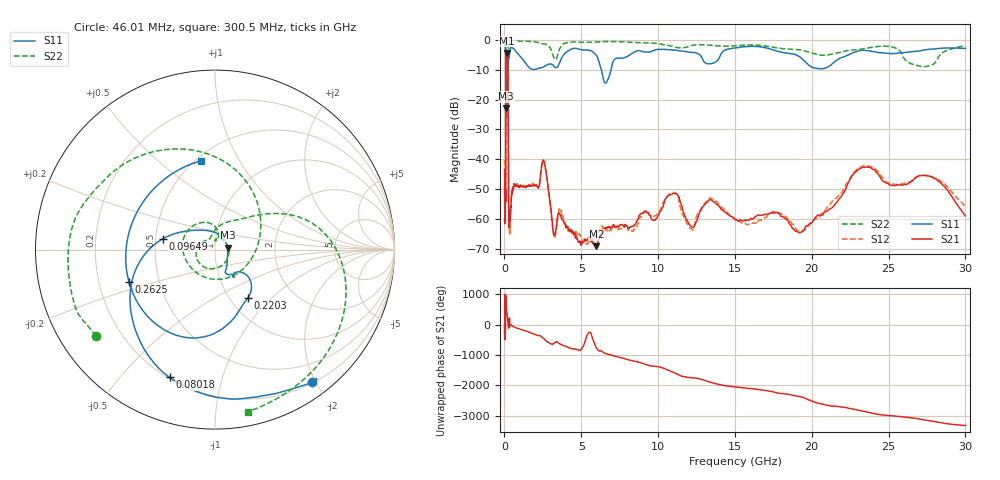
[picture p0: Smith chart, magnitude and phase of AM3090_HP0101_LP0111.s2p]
! Date/Time: Thu, Feb 28, 2019 1:58 PM
! Network Analyzer: Agilent Technologies E8364B Rev: A.07.50.67
! Sweep from 0.010 to 30.000 GHz, 1601 Points, Sweep Type: LOG
! Power Supply: 5.023 V, 0.002 A
# Hz S DB R 50
!freq MagS11 AngS11 MagS21 AngS21 MagS12 AngS12 MagS22 AngS22
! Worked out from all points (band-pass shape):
!   1601 points, 10 MHz to 30 GHz, reference 50 ohm
!   highest |S21| = -4.35 dB at 155.2 MHz (marker M1); lowest = -69.2 dB at 5.989 GHz (marker M2)
!   |S21| within 3 dB of the highest: 107.8 MHz to 217.4 MHz (109.6 MHz wide, 67.4 % of centre)
!   lowest |S11| = -23.0 dB at 105.1 MHz (marker M3), VSWR 1.15, Z = 57.5 + j1.26 ohm
!   |S11| at or under -10 dB: 96.1 MHz to 217.8 MHz (121.7 MHz wide, 77.5 % of centre); 6.308 GHz to 6.931 GHz (622.9 MHz wide, 9.41 % of centre)
!   |S22| runs from -26.4 to -0.2 dB; largest |S21 - S12| = 0.014
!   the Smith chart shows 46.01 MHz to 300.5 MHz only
!   S11 on the Smith chart (normalised r, x): 46.01 MHz: 0.21, -1.95; 80.18 MHz: 0.21, -0.69; 96.49 MHz: 0.55, +0.07; 220.3 MHz: 1.20, -0.73; 262.5 MHz: 0.33, -0.16; 300.5 MHz: 0.53, +0.71
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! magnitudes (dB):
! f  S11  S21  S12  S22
! 10 MHz  -0.3  -43.4  -40.2  -0.5
! 38.04 MHz  -0.5  -59.4  -60.0  -1.4
! 46.01 MHz  -0.8  -53.6  -50.1  -1.7
! 80.18 MHz  -2.4  -50.2  -49.3  -4.8
! 96.49 MHz  -10.6  -16.6  -16.6  -15.6
! 105.1 MHz  -23.0  -8.3  -8.4  -14.6
! 144.7 MHz  -15.9  -4.4  -4.4  -23.2
! 155.2 MHz  -15.5  -4.4  -4.3  -21.5
! 220.3 MHz  -9.7  -7.9  -7.9  -15.0
! 262.5 MHz  -5.8  -48.4  -50.2  -1.7
! 300.5 MHz  -6.0  -59.6  -62.3  -0.7
! 550.5 MHz  -2.8  -50.0  -49.4  -0.3
! 2.084 GHz  -9.8  -48.7  -49.1  -0.7
! 2.558 GHz  -8.9  -40.6  -40.5  -1.3
! 3.22 GHz  -8.8  -65.4  -64.9  -6.1
! 5.989 GHz  -5.2  -69.2  -65.5  -0.7
! 7.926 GHz  -5.7  -62.2  -62.2  -0.7
! 10.86 GHz  -3.3  -51.8  -51.4  -2.0
! 12.01 GHz  -4.1  -61.7  -62.5  -2.1
! 19.51 GHz  -7.0  -63.7  -63.7  -3.6
! 23.48 GHz  -3.5  -42.7  -42.2  -2.9
! 30 GHz  -2.9  -59.1  -56.0  -2.1
